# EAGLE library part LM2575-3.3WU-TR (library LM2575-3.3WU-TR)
Switching Voltage Regulators Source: Datasheet
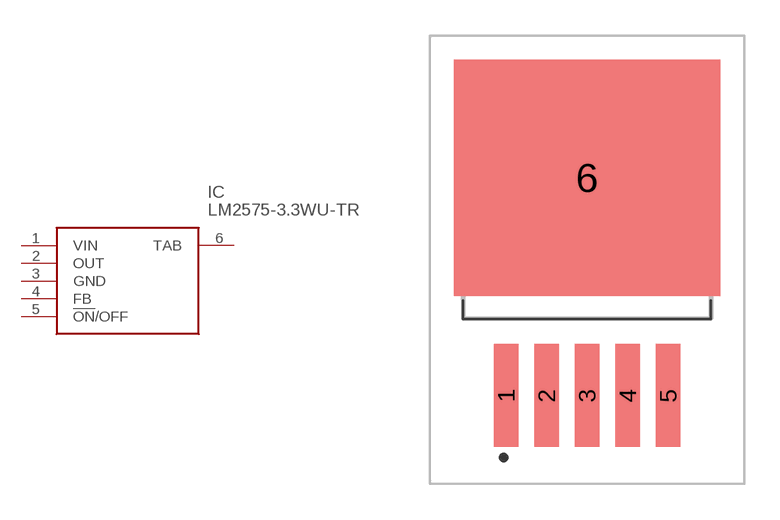
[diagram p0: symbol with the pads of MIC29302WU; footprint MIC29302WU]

Designator prefix IC

## LM2575-3.3WU-TR (Description: Switching Voltage Regulators; Height: 4mm; Manufacturer_Name: Microchip; Manufacturer_Part_Number: LM2575-3.3WU-TR; Mouser_Part_Number: 998-LM2575-3.3WUTR; Mouser_Price-Stock: https://www.mouser.co.uk/ProductDetail/Microchip-Technology/LM2575-3.3WU-TR?qs=Y3Q3JoKAO1TNQ1s9ijuGrQ%3D%3D)  [MIC29302WU]
1  VIN
2  OUT
3  GND
4  FB
5  !ON!/OFF
6  TAB

## Footprint MIC29302WU (pad centres in mm)
5-Lead TO-263
smd 1.02 x 4.32: 1 -3.4,-12; 2 -1.7,-12; 3 0,-12; 4 1.7,-12; 5 3.4,-12
smd 11.18 x 9.91: 6 0,-2.855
